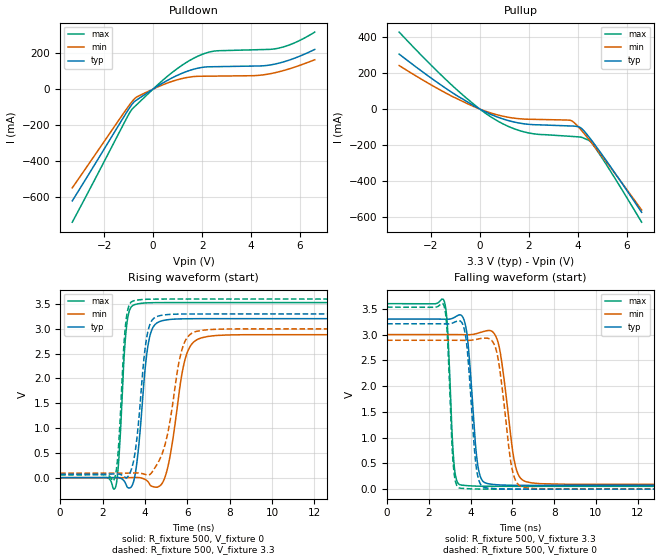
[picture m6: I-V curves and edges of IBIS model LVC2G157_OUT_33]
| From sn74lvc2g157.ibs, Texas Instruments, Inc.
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[Model]   LVC2G157_OUT_33
Model_type  Output
Vref =   0
Rref =   500
Cref =   50p
Vmeas =   1.5
| variable   typ   min   max
C_comp   9.43pF   5.87pF   12.80pF
| C_pullup   9.59pF   5.87pF   11.73pF
| C_pulldown   9.26pF   6.39pF   12.80pF
[Temperature Range]   40   100   -40
| Ambient temperature   25   85   -40
[Voltage range]   3.3   3   3.6
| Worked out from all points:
|   slope of the pulldown table from 0 to 0.495 V, typ, clamps not added: 11.9 ohm
|   slope of the pullup table from 0 to 0.495 V, typ, clamps not added: 15.5 ohm
|   rising waveform, R_fixture 500, V_fixture 0: 20-80 % time 403ps typ, 604ps min, 265ps max; typ from 0 V to 3.21 V
|   falling waveform, R_fixture 500, V_fixture 3.3: 20-80 % time 353ps typ, 532ps min, 232ps max; typ from 3.3 V to 0.073 V
|   rising waveform, R_fixture 500, V_fixture 3.3: 20-80 % time 423ps typ, 698ps min, 270ps max; typ from 0.073 V to 3.3 V
|   falling waveform, R_fixture 500, V_fixture 0: 20-80 % time 341ps typ, 508ps min, 223ps max; typ from 3.21 V to 0 V
[Pulldown]
| LVC2G157_OUT_33
|   Voltage   I(typ)   I(min)   I(max)
-3.3V     -624.5mA   -551.6mA   -743.5mA
-910mV    -94.39mA   -78.81mA   -121.9mA
-785mV    -73.05mA   -57.97mA   -102.4mA
-625mV    -56.69mA   -41.11mA   -81.37mA
775mV     62.29mA    42.84mA    92.23mA
1.545V    106.3mA    68.02mA    163.8mA
2.23V     124.1mA    71.96mA    204.2mA
2.635V    125.2mA    72.54mA    213.9mA
4.185V    128.6mA    75.28mA    219.5mA
5.06V     142.2mA    93.97mA    226.8mA
5.775V    172.4mA    122.4mA    258.2mA
6.6V      221.3mA    163.7mA    318.2mA
[Pullup]
| LVC2G157_OUT_33
|   Voltage   I(typ)   I(min)   I(max)
-3.3V     305.1mA    241.7mA    427.2mA
-1.05V    84.45mA    65.23mA    120.7mA
-50mV     3.654mA    2.736mA    5.316mA
595mV     -37.54mA   -27.41mA   -55.66mA
1.255V    -66.83mA   -47.19mA   -101.2mA
1.92V     -83.22mA   -55.82mA   -130mA
3.76V     -93.58mA   -66.15mA   -151.3mA
4.12V     -104.2mA   -113.9mA   -155.3mA
4.445V    -153.3mA   -167.1mA   -173.4mA
4.565V    -174.5mA   -187.6mA   -188.3mA
5.3V      -313mA     -318.2mA   -337.6mA
6.6V      -571.9mA   -558.9mA   -626.7mA
[Ramp]
| LVC2G157_OUT_33
| variable   typ   min   max
dV/dt_r   2.05/4.36E-10   1.85/6.51E-10   2.26/2.89E-10
dV/dt_f   1.99/3.72E-10   1.79/5.53E-10   2.18/2.47E-10
R_load = 500
[Rising Waveform]
| LVC2G157_OUT_33
R_fixture =   500
C_fixture =   0
L_fixture =   0
V_fixture =   0
V_fixture_min = 0
V_fixture_max = 0
|   Time   V(typ)   V(min)   V(max)
0s        146.9pV    5.297nV    581.1pV
2.6ns     2.207mV    -60.71uV   -207.1mV
2.77ns    816.4uV    -36.41uV   376.4mV
3.13ns    -156.1mV   411.9uV    3.033V
3.55ns    90.27mV    3.551mV    3.492V
4.16ns    2.699V     -87.45mV   3.525V
4.775ns   3.158V     -137.6mV   3.529V
5.9ns     3.202V     2.391V     3.529V
6.665ns   3.204V     2.818V     3.529V
27ns      3.205V     2.883V     3.529V
[Falling Waveform]
| LVC2G157_OUT_33
R_fixture =   500
C_fixture =   0
L_fixture =   0
V_fixture =   3.3
V_fixture_min = 3
V_fixture_max = 3.6
|   Time   V(typ)   V(min)   V(max)
0s        3.3V       3V         3.6V
2.73ns    3.298V     3V         3.657V
3.2ns     3.328V     3V         530.1mV
3.475ns   3.383V     2.999V     88.61mV
3.84ns    2.977V     2.997V     68.58mV
4.355ns   439.9mV    3.027V     58.31mV
4.755ns   114.6mV    3.072V     56.2mV
5.325ns   84.07mV    2.838V     55.29mV
6.655ns   73.43mV    144.6mV    55mV
27ns      72.55mV    92mV       54.93mV
[Rising Waveform]
| LVC2G157_OUT_33
R_fixture =   500
C_fixture =   0
L_fixture =   0
V_fixture =   3.3
V_fixture_min = 3
V_fixture_max = 3.6
|   Time   V(typ)   V(min)   V(max)
0s        72.51mV    91.94mV    54.9mV
2.55ns    74.03mV    91.88mV    -33.66mV
2.745ns   75.13mV    91.91mV    565.1mV
3.085ns   1.618mV    92.24mV    3.071V
3.46ns    324.2mV    94.42mV    3.564V
4.085ns   2.824V     57.62mV    3.596V
4.62ns    3.256V     302.2mV    3.599V
5.75ns    3.298V     2.582V     3.6V
6.42ns    3.3V       2.948V     3.6V
27ns      3.3V       3V         3.6V
[Falling Waveform]
| LVC2G157_OUT_33
R_fixture =   500
C_fixture =   0
L_fixture =   0
V_fixture =   0
V_fixture_min = 0
V_fixture_max = 0
|   Time   V(typ)   V(min)   V(max)
0s        3.209V     2.89V      3.532V
2.715ns   3.208V     2.89V      3.573V
3.17ns    3.229V     2.89V      480.1mV
3.46ns    3.269V     2.889V     22.34mV
3.815ns   2.809V     2.887V     10.71mV
4.29ns    374mV      2.907V     2.968mV
4.67ns    33.3mV     2.93V      1.178mV
5.235ns   8.643mV    2.69V      360.7uV
6.48ns    713.5uV    41.76mV    92.29uV
27ns      35.38uV    50.86uV    25.66uV
